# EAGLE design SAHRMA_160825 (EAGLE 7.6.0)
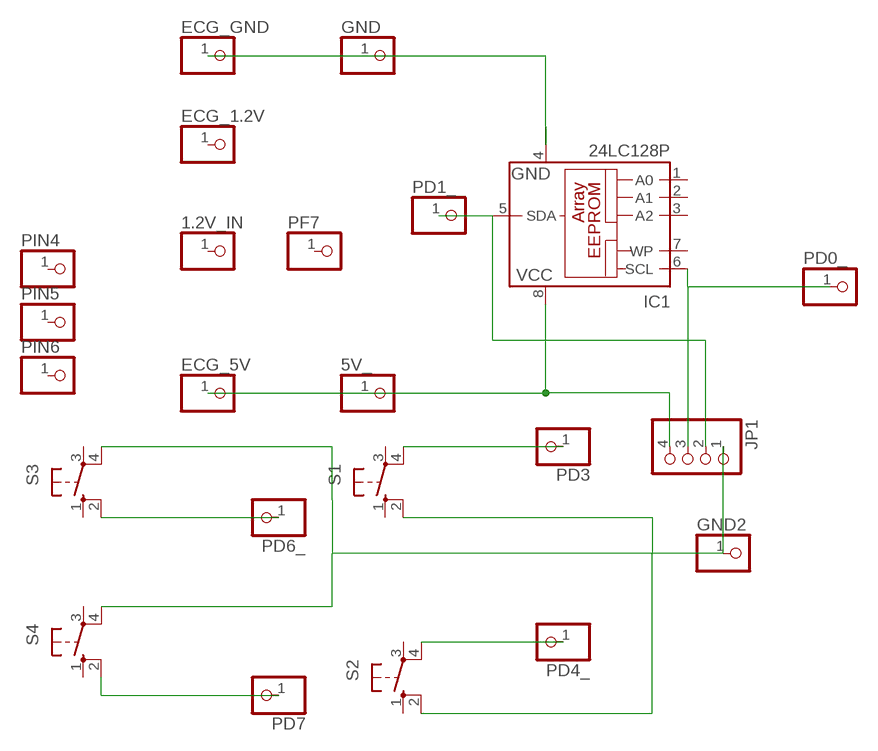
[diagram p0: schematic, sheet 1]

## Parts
1.2V_IN  PINHD-1X1  [1X01]
5V_  PINHD-1X1  [1X01]
ECG_1.2V  PINHD-1X1  [1X01]
ECG_5V  PINHD-1X1  [1X01]
ECG_GND  PINHD-1X1  [1X01]
GND  PINHD-1X1  [1X01]
GND2  PINHD-1X1  [1X01]
IC1  24LC128P  [DIL8]
JP1  PINHD-1X4  [1X04]
PD0_  PINHD-1X1  [1X01]
PD1_  PINHD-1X1  [1X01]
PD3  PINHD-1X1  [1X01]
PD4_  PINHD-1X1  [1X01]
PD6_  PINHD-1X1  [1X01]
PD7  PINHD-1X1  [1X01]
PF7  PINHD-1X1  [1X01]
PIN4  PINHD-1X1  [1X01]
PIN5  PINHD-1X1  [1X01]
PIN6  PINHD-1X1  [1X01]
S1  10-XX  [B3F-10XX]
S2  10-XX  [B3F-10XX]
S3  10-XX  [B3F-10XX]
S4  10-XX  [B3F-10XX]

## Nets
N$1: IC1.5(SDA) JP1.2 PD1_.1
N$2: 5V_.1 ECG_5V.1 IC1.8(VCC) JP1.4
N$3: IC1.6(SCL) JP1.3 PD0_.1
N$4: ECG_GND.1 GND.1 IC1.4(GND)
N$5: PD3.1 S1.4(P1)
N$8: PD7.1 S4.2(S1)
N$9: GND2.1 JP1.1 S1.2(S1) S2.2(S1) S3.4(P1) S4.4(P1)
N$10: PD4_.1 S2.4(P1)
N$11: PD6_.1 S3.2(S1)
Unconnected: 1.2V_IN.1 ECG_1.2V.1 IC1.1(A0) IC1.2(A1) IC1.3(A2) IC1.7(WP) PF7.1 PIN4.1 PIN5.1 PIN6.1 S1.1(S) S1.3(P) S2.1(S) S2.3(P) S3.1(S) S3.3(P) S4.1(S) S4.3(P)

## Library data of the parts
1.2V_IN 5V_ ECG_1.2V ECG_5V ECG_GND GND GND2 PD0_ PD1_ PD3 PD4_ PD6_ PD7 PF7 PIN4-PIN6 = pinhead:PINHD-1X1: PIN HEADER
IC1 = microchip:24*: Serial EEPROM I2C; MF: MICROCHIP; MPN: 24LC128-I/P; OC_FARNELL: 9757929; OC_NEWARK: 12C2007
JP1 = pinhead:PINHD-1X4: PIN HEADER
S1-S4 = switch-omron:10-XX: OMRON SWITCH; MPN: B3F-1000; OC_FARNELL: 176432; OC_NEWARK: 36M3542

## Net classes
0 default: width 0.406 mm

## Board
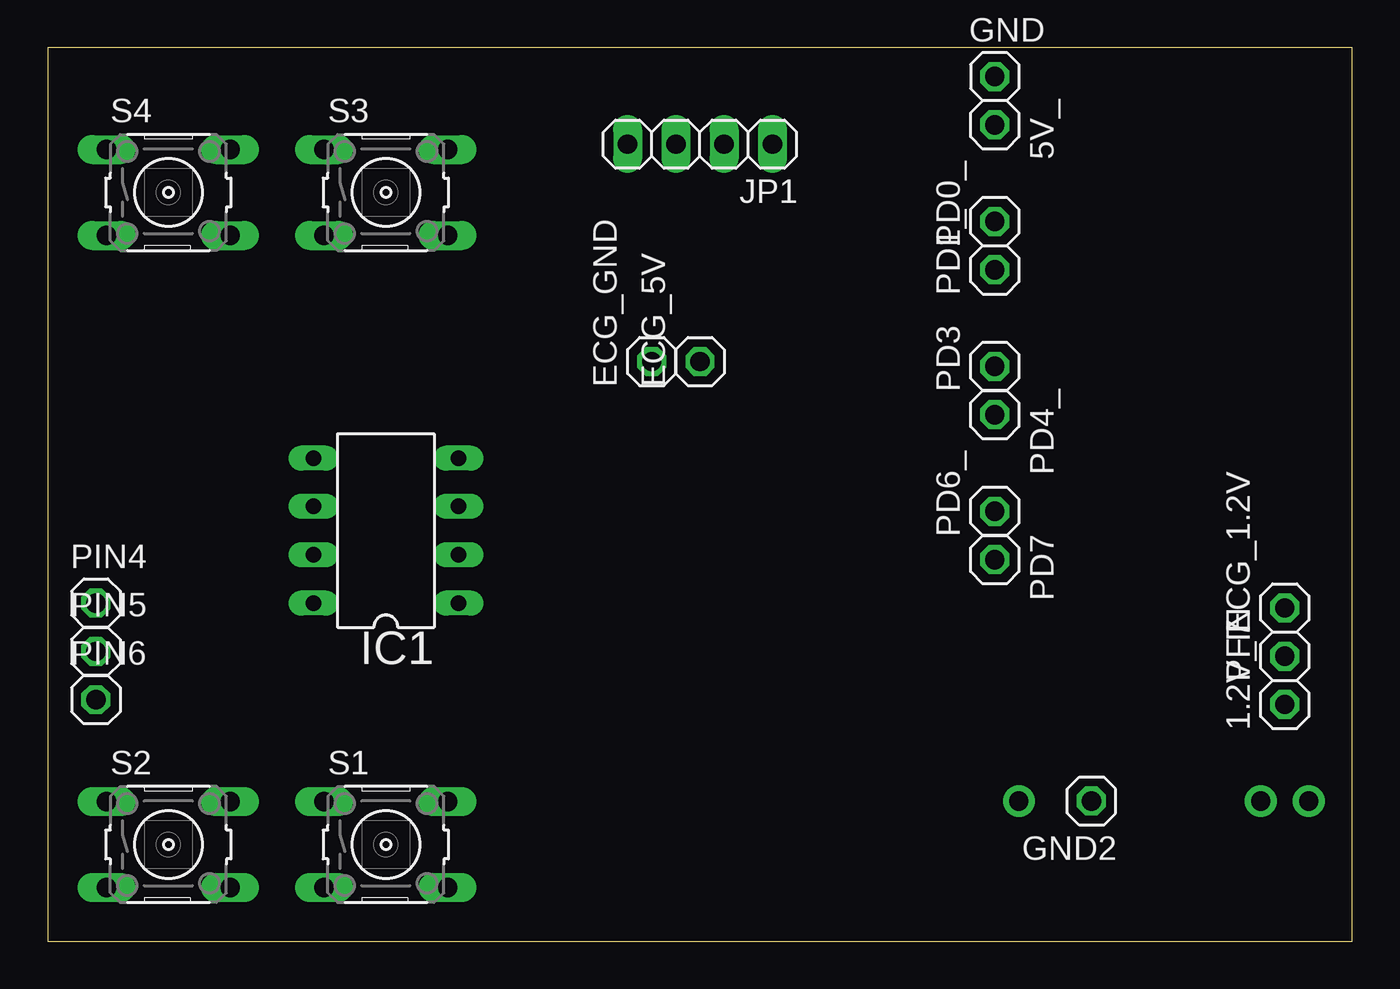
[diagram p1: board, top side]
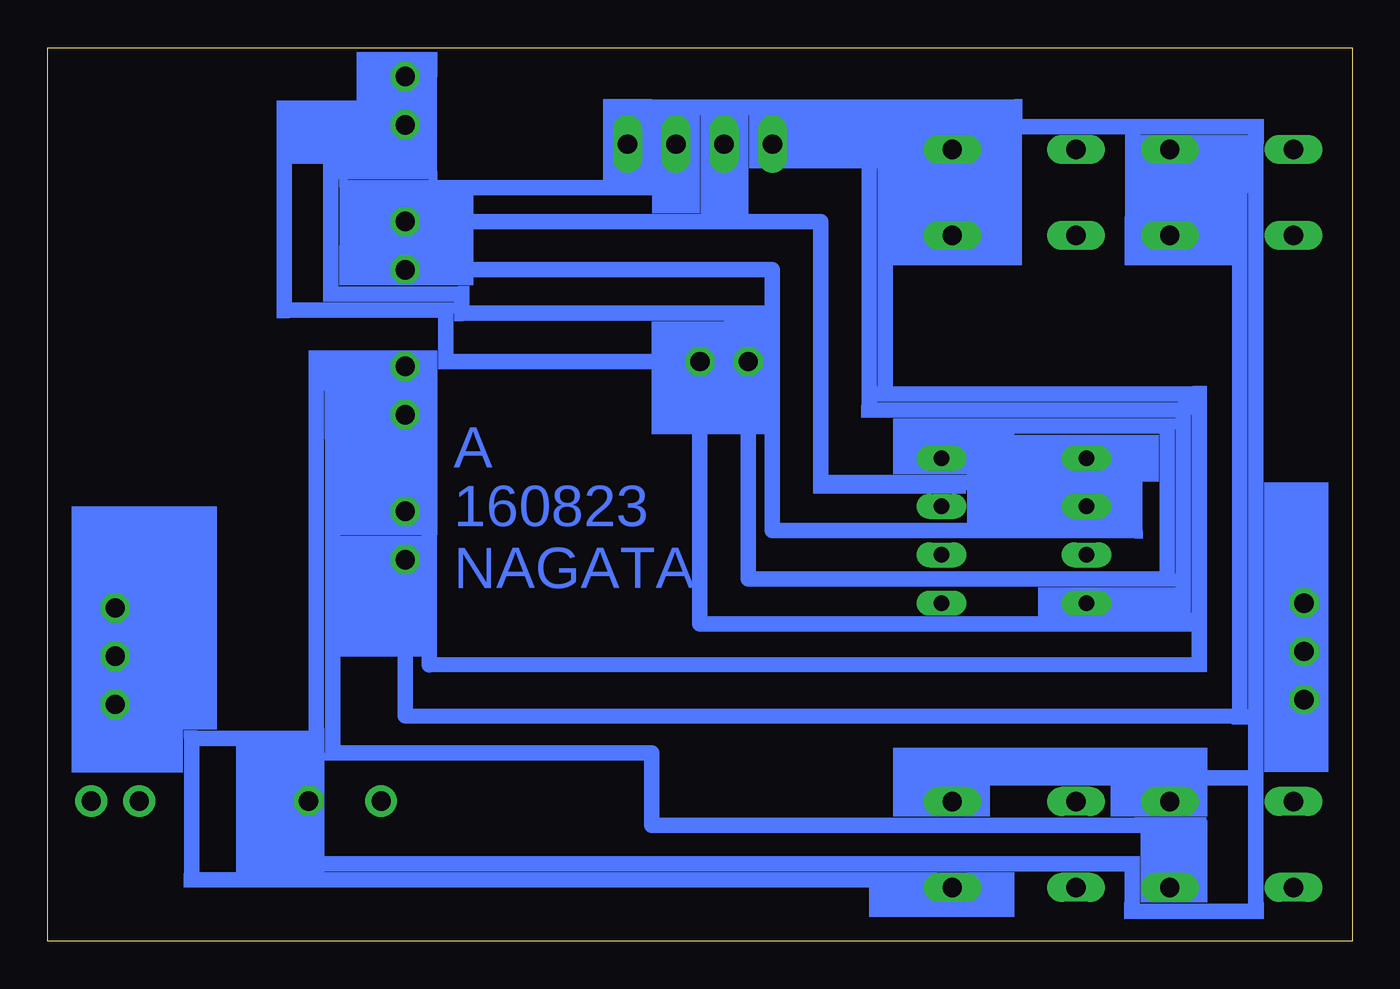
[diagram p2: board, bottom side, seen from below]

Size 68.58 x 46.99 mm. Coordinates in mm from the lower left corner, seen from the top.
Outline: 0,0 68.58,0 68.58,46.99 0,46.99 0,0
Copper layers (1*16): Top 0.035mm / dielectric 1.5mm / Bottom 0.035mm
Design rules "default *": minimum track width 32mil, minimum drill 24mil, track to track 8mil, track to pad 8mil, pad to pad 8mil, via to via 8mil, smd to smd 8mil, copper to edge 40mil, drill to drill 8mil, minimum pad ring 10mil, minimum via ring 8mil, stop-mask expansion 4mil, vias tented up to drill 0mil, thermal gap 10mil

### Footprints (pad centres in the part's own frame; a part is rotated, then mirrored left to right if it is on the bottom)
1X01 = drill 1.016 octagon: 1 0,0
DIL8 = drill 0.813 long: 1 -3.81,-3.81; 2 -1.27,-3.81; 3 1.27,-3.81; 4 3.81,-3.81; 5 3.81,3.81; 6 1.27,3.81; 7 -1.27,3.81; 8 -3.81,3.81
1X04 = drill 1.016 long: 1 -3.81,0; 2 -1.27,0; 3 1.27,0; 4 3.81,0
B3F-10XX = drill 1.016 long: 1 -3.251,2.261; 2 3.251,2.261; 3 -3.251,-2.261; 4 3.251,-2.261

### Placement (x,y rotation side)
1.2V_IN  65.02,12.45 90 top
5V_  49.78,42.93 270 top
ECG_1.2V  65.02,17.53 90 top
ECG_5V  34.29,30.48 90 top
ECG_GND  31.75,30.48 90 top
GND  49.78,45.47 0 top
GND2  54.86,7.37 180 top
IC1  17.78,21.59 90 top
JP1  34.29,41.91 180 top
PD0_  49.78,37.85 90 top
PD1_  49.78,35.31 90 top
PD3  49.78,30.23 90 top
PD4_  49.78,27.69 270 top
PD6_  49.78,22.61 90 top
PD7  49.78,20.07 270 top
PF7  65.02,14.99 90 top
PIN4  2.54,17.78 0 top
PIN5  2.54,15.24 0 top
PIN6  2.54,12.7 0 top
S1  17.78,5.08 0 top
S2  6.35,5.08 0 top
S3  17.78,39.37 0 top
S4  6.35,39.37 0 top

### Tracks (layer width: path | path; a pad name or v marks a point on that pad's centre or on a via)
N$1
  Bottom 0.813: IC1.5 11.43,25.4 11.43,21.59 30.48,21.59 30.48,35.31 PD1_.1 52.83,35.31 52.83,39.62 35.56,39.62 JP1.2
N$2
  Bottom 0.813: JP1.4 25.4,41.91 25.4,27.94 8.89,27.94 8.89,16.69 13.97,16.69 | 13.97,16.69 34.29,16.69 ECG_5V.1 47.65,30.48 47.65,33.17 56.13,33.17 56.13,42.93 5V_.1 | 13.97,16.69 IC1.8
N$3
  Bottom 0.813: JP1.3 33.02,37.85 | 33.02,37.85 PD0_.1 | 33.02,37.85 27.94,37.85 27.94,24.13 19.05,24.13 19.05,22.86 IC1.6
N$4
  Bottom 0.813: IC1.4 21.59,27.08 9.73,27.08 9.73,19.05 31.75,19.05 ECG_GND.1 31.75,33.02 46.81,33.02 46.81,34.04 53.7,34.04 53.7,40.46 48.51,40.46 48.51,45.47 GND.1
N$5
  Bottom 0.813: PD3.1 54.46,30.23 54.46,10.67 61.01,10.67 61.01,3.23 21.03,3.23 S1.4
N$8
  Bottom 0.813: S4.2 5.92,41.63 5.92,11.81 49.78,11.84 PD7.1
N$9
  Bottom 0.813: 5.08,8.59 5.08,42.82 11.56,42.82 | 9.6,8.59 21.03,8.59 S1.2 | 5.08,8.59 9.6,8.59 | 9.6,8.59 S2.2 | GND2.1 54.86,4.06 11.58,4.06 11.58,1.57 5.08,1.57 5.08,8.59 | S4.4 11.56,37.11 11.56,42.82 | S3.4 17.78,37.11 17.78,42.82 | 17.78,42.82 11.56,42.82 | JP1.1 38.1,43.87 17.75,43.87 17.78,42.82
N$10
  Bottom 0.813: PD4_.1 53.59,27.69 53.59,9.91 36.83,9.91 36.83,6.1 9.6,6.1 S2.4
N$11
  Bottom 0.813: S3.2 24.56,41.63 24.56,28.78 8.05,28.78 8.05,14.55 48.51,14.53 48.51,22.61 PD6_.1
N$14  (via drill 1 pad 1.68)
  other vias: 51.05,7.37
N$19  (via drill 1 pad 1.68)
  other vias: 63.75,7.37
N$20  (via drill 1 pad 1.68)
  other vias: 66.29,7.37
(copper drawn outside any net)
  shapes: Bottom area x133

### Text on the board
Bottom: A | 160823 / NAGATA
